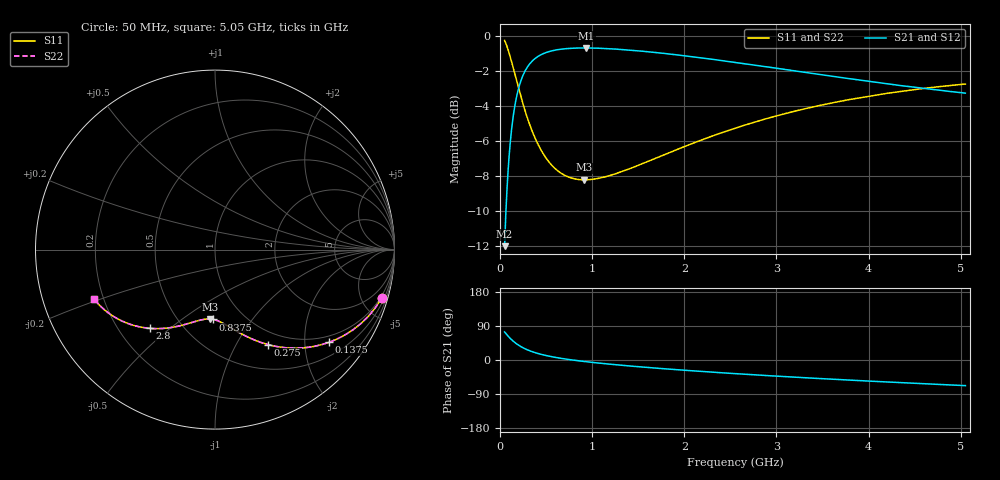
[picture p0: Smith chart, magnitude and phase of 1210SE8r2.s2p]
! AVX Thin Film Operation		Date: August 2001
! Description: Accu-P® Series, Thin Film, SMD, RF Capacitor
! Part Number: 12101J8R2BBT
! 50 MHz  -  5.05 GHz
! Serial Measurements
# mhz S db R 50
!	S11		S21		S12		S22
!	dB	Phase	dB	Phase	dB	Phase	dB	Phase
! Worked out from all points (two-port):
!   401 points, 50 MHz to 5.05 GHz, reference 50 ohm
!   highest |S21| = -0.71 dB at 937.5 MHz (marker M1); lowest = -12.0 dB at 50 MHz (marker M2)
!   |S21| within 3 dB of the highest: 171.7 MHz to end of sweep
!   lowest |S11| = -8.2 dB at 912.5 MHz (marker M3), VSWR 2.27, Z = 35.3 - j32.2 ohm
!   |S11| at or under -10 dB: nowhere
!   |S22| runs from -8.2 to -0.3 dB; largest |S21 - S12| = 0
!   S11 on the Smith chart (normalised r, x): 50 MHz: 0.83, -7.02; 137.5 MHz: 0.82, -2.59; 275 MHz: 0.81, -1.36; 837.5 MHz: 0.72, -0.66; 2.8 GHz: 0.33, -0.43; 5.05 GHz: 0.16, -0.19
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50  -0.28 -16.0  -12.01 74.0  -12.01 74.0  -0.28 -16.0
75  -0.61 -23.4  -8.85 66.6  -8.85 66.6  -0.61 -23.4
100  -1.02 -30.1  -6.81 59.9  -6.81 59.9  -1.02 -30.1
137.5  -1.73 -39.0  -4.84 51.0  -4.84 51.0  -1.73 -39.0
162.5  -2.23 -44.1  -3.97 45.9  -3.97 45.9  -2.23 -44.1
200  -2.98 -50.7  -3.05 39.3  -3.05 39.3  -2.98 -50.7
275  -4.34 -60.8  -1.99 29.2  -1.99 29.2  -4.34 -60.8
362.5  -5.62 -69.1  -1.39 20.8  -1.39 20.8  -5.62 -69.1
487.5  -6.89 -77.5  -0.99 12.5  -0.99 12.5  -6.89 -77.5
637.5  -7.76 -84.6  -0.80 5.4  -0.80 5.4  -7.76 -84.6
837.5  -8.20 -91.6  -0.71 -1.6  -0.71 -1.6  -8.20 -91.6
887.5  -8.22 -93.1  -0.71 -3.1  -0.71 -3.1  -8.22 -93.1
912.5  -8.23 -93.8  -0.71 -3.9  -0.71 -3.9  -8.23 -93.8
937.5  -8.23 -94.5  -0.71 -4.6  -0.71 -4.6  -8.23 -94.5
1312.5  -7.78 -103.7  -0.80 -13.8  -0.80 -13.8  -7.78 -103.7
1725  -6.92 -112.0  -0.99 -22.1  -0.99 -22.1  -6.92 -112.0
2125  -6.08 -119.1  -1.23 -29.2  -1.23 -29.2  -6.08 -119.1
2550  -5.29 -126.0  -1.53 -36.0  -1.53 -36.0  -5.29 -126.0
2800  -4.88 -129.7  -1.72 -39.7  -1.72 -39.7  -4.88 -129.7
3387.5  -4.08 -137.9  -2.16 -47.9  -2.16 -47.9  -4.08 -137.9
4225  -3.28 -148.3  -2.77 -58.3  -2.77 -58.3  -3.28 -148.3
5050  -2.77 -157.6  -3.29 -67.6  -3.29 -67.6  -2.77 -157.6
